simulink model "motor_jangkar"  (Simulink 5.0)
settings: Solver=ode4  StartTime=0.0  StopTime=5  FixedStep=0.001  RelTol=1e-6
libraries: simulink x3

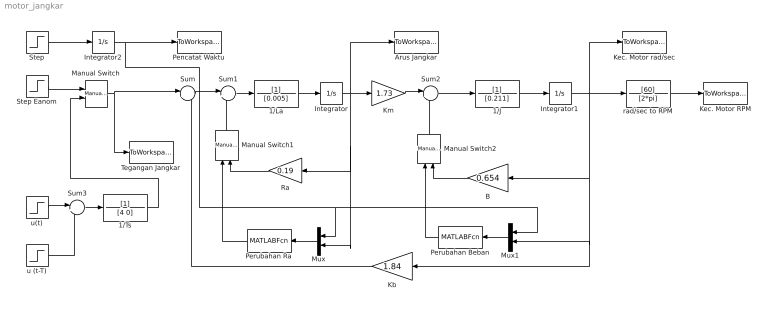
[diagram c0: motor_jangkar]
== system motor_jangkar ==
  1/J : TransferFcn  Denominator=[0.211]
  1/La : TransferFcn  Denominator=[0.005]
  1/Ts : TransferFcn  Denominator=[4 0]
  Arus Jangkar : ToWorkspace  VariableName=arus  SampleTime=-1  SaveFormat=Array
  B : Gain  Orientation=left  Gain=0.654
  Integrator : Integrator
  Integrator1 : Integrator
  Integrator2 : Integrator
  Kb : Gain  Orientation=left  Gain=1.84
  Kec. Motor RPM : ToWorkspace  VariableName=rpm  SampleTime=-1  SaveFormat=Array
  Kec. Motor rad/sec : ToWorkspace  VariableName=omega  SampleTime=-1  SaveFormat=Array
  Km : Gain  Gain=1.73
  Manual Switch : simulink/Signal Routing/Manual Switch  sw=0  action=0
  Manual Switch1 : simulink/Signal Routing/Manual Switch  Orientation=up  sw=0  action=0
  Manual Switch2 : simulink/Signal Routing/Manual Switch  Orientation=up  sw=0  action=0
  Mux : Mux  Orientation=left  Inputs=2
  Mux1 : Mux  Orientation=left  Inputs=2
  Pencatat Waktu : ToWorkspace  VariableName=time  SampleTime=-1  SaveFormat=Array
  Perubahan Beban : MATLABFcn  Orientation=left  MATLABFcn=variasi_beban
  Perubahan Ra : MATLABFcn  Orientation=left  MATLABFcn=variasi_r
  Ra : Gain  Orientation=left  Gain=0.19
  Step : Step  Time=0  SampleTime=0
  Step Eanom : Step  Time=0.01  After=500  SampleTime=0
  Sum{,1..3} (4 alike) : Sum  Inputs=|+-
  Tegangan Jangkar : ToWorkspace  VariableName=tegangan  SampleTime=-1  SaveFormat=Array
  rad/sec to RPM : TransferFcn  Numerator=[60]  Denominator=[2*pi]
  u (t-T) : Step  Time=4  After=500  SampleTime=0
  u(t) : Step  Time=0  After=500  SampleTime=0
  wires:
  Step/1 -> Integrator2/1
  Integrator2/1 -> Pencatat Waktu/1, Mux/1, Mux1/1
  Sum/1 -> Sum1/1
  Sum1/1 -> 1/La/1
  1/La/1 -> Integrator/1
  Integrator/1 -> Km/1, Arus Jangkar/1, Ra/1, Mux/2
  Km/1 -> Sum2/1
  Sum2/1 -> 1/J/1
  1/J/1 -> Integrator1/1
  Integrator1/1 -> rad/sec to RPM/1, B/1, Kb/1, Mux1/2, Kec. Motor rad/sec/1
  Kb/1 -> Sum/2
  rad/sec to RPM/1 -> Kec. Motor RPM/1
  Step Eanom/1 -> Manual Switch/1
  Manual Switch/1 -> Sum/1, Tegangan Jangkar/1
  u(t)/1 -> Sum3/1
  u (t-T)/1 -> Sum3/2
  Sum3/1 -> 1/Ts/1
  Mux/1 -> Perubahan Ra/1
  Manual Switch1/1 -> Sum1/2
  Perubahan Ra/1 -> Manual Switch1/1
  Ra/1 -> Manual Switch1/2
  Mux1/1 -> Perubahan Beban/1
  Manual Switch2/1 -> Sum2/2
  Perubahan Beban/1 -> Manual Switch2/1
  B/1 -> Manual Switch2/2
  1/Ts/1 -> Manual Switch/2
